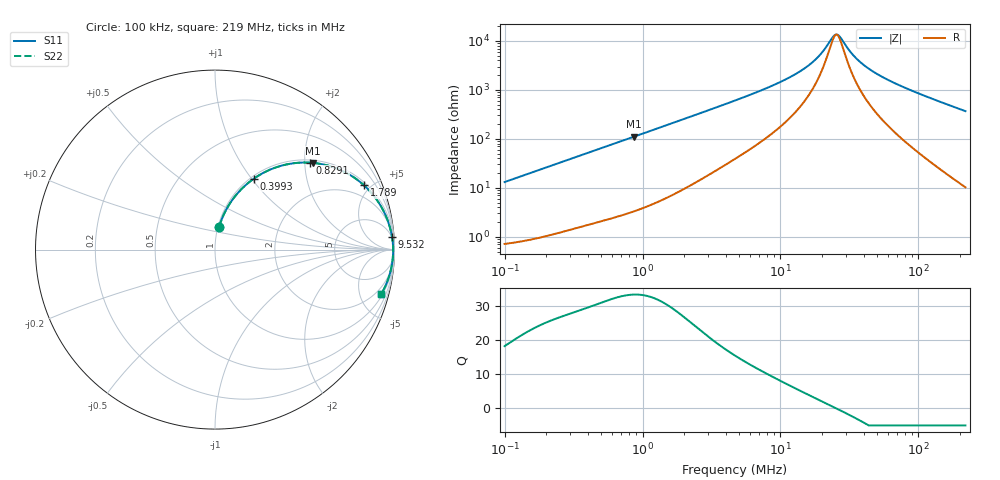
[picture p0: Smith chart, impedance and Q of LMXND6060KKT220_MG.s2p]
! LMXND6060KKT220_MG  S-PARAMETER MODEL  ( General Type )
! Model Generated by TAIYO YUDEN Corporation (http://www.ty-top.com)
! Version 1.0
! TAIYO YUDEN Control No. 191023NI43SB-FBB
! Copyright(c) 2019 TAIYO YUDEN CO.,LTD. All Rights Reserved.
! Product Description (link to TY-COMPAS)
! https://ds.yuden.co.jp/TYCOMPAS/or/detail?pn=LMXND6060KKT220MMG&u=M
! Products Name : Inductors
! Characteristics :
!  Inductance : 22 uH , SRF(min) : 12 MHz , DC Resistance(max) : 0.696 Ohm
!  Rated Current : Saturation :650 mA , Temp Rise : 700 mA
!  Case Size : 6.0 x 6.0 / 0.236 x 0.236 [mm/inch] , Thickness : 1 / 0.039 [mm/inch]
!  (Conditions: Temperature = 25 degC , DC Bias Current/Voltage = 0A / 0V)
! External Node Assignments :
!  1  o---GGG---o  2
! GND o---------o GND
! Frequency Range : 0.1MHz  -  218.972167MHz  [ 402 STEP ]
# MHz S RI R 50
! Freq[MHz].  S11 Real  S11 Imag  S21 Real  S21 Imag  S12 Real  S12 Imag  S22 Real  S22 Imag
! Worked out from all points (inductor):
!   401 points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, 100 kHz to 219 MHz, reference 50 ohm
!   read as one part in series: L = 20.8 uH near 103.9 kHz
!   highest Q = 33.5 at 861.6 kHz (marker M1), where L = 20.3 uH
!   self-resonance near 25.41 MHz
!   S11 on the Smith chart (normalised r, x): 100 kHz: 1.01, +0.26; 399.3 kHz: 1.03, +1.03; 829.1 kHz: 1.06, +2.12; 1.789 MHz: 1.16, +4.56; 9.532 MHz: 4, +27; 219 MHz: 1.21, -7.36
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0.1  0.0236 0.127  0.9764 -0.127  0.9764 -0.127  0.0236 0.127
0.207652  0.0765 0.247  0.9235 -0.247  0.9235 -0.247  0.0765 0.247
0.362673  0.1881 0.374  0.8119 -0.374  0.8119 -0.374  0.1881 0.374
0.399273  0.2173 0.3959  0.7827 -0.3959  0.7827 -0.3959  0.2173 0.3959
0.8291  0.5279 0.4845  0.4721 -0.4845  0.4721 -0.4845  0.5279 0.4845
0.861606  0.5463 0.4831  0.4537 -0.4831  0.4537 -0.4831  0.5463 0.4831
1.315317  0.7311 0.4279  0.2689 -0.4279  0.2689 -0.4279  0.7311 0.4279
1.789146  0.8301 0.3584  0.1699 -0.3584  0.1699 -0.3584  0.8301 0.3584
2.784314  0.9169 0.2543  0.0831 -0.2543  0.0831 -0.2543  0.9169 0.2543
4.770297  0.965 0.1541  0.035 -0.1541  0.035 -0.1541  0.965 0.1541
9.531921  0.9864 0.0711  0.0136 -0.0711  0.0136 -0.0711  0.9864 0.0711
13.21743  0.9902 0.0439  0.00983 -0.0439  0.00983 -0.0439  0.9902 0.0439
16.97108  0.9917 0.0261  0.00828 -0.0261  0.00828 -0.0261  0.9917 0.0261
19.79326  0.9923 0.0159  0.00772 -0.0159  0.00772 -0.0159  0.9923 0.0159
23.98983  0.9926 0.00368  0.00737 -0.00368  0.00737 -0.00368  0.9926 0.00368
25.90783  0.9927 -0.00116  0.00732 0.00116  0.00732 0.00116  0.9927 -0.00116
33.26547  0.9925 -0.0171  0.00753 0.0171  0.00753 0.0171  0.9925 -0.0171
38.05839  0.9921 -0.026  0.00789 0.026  0.00789 0.026  0.9921 -0.026
47.02309  0.9911 -0.0411  0.00888 0.0411  0.00888 0.0411  0.9911 -0.0411
61.54953  0.9888 -0.0629  0.0112 0.0629  0.0112 0.0629  0.9888 -0.0629
107.4986  0.9771 -0.1237  0.0229 0.1237  0.0229 0.1237  0.9771 -0.1237
218.9722  0.9253 -0.2493  0.0747 0.2493  0.0747 0.2493  0.9253 -0.2493
